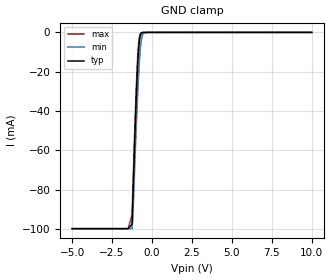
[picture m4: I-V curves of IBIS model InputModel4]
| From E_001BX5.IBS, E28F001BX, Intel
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|*******************Input Model 4************************************
[Model]   InputModel4
Model_type   Input
|   Model for pin A[10]
Vinl = 0.8V
Vinh = 2.0V
|Variable   Typ   Min   Max
C_comp   9.13p   7.20p   11.06p
[Voltage Range]   5.0V   4.5V   5.5V
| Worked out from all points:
|   GND clamp passes 1 mA (typ) near -0.71 V on its own axis
[GND_clamp]
|Voltage   I(typ)   I(min)   I(max)
-5V       -99.85mA   -99.85mA   -99.85mA
-1.5V     -99.85mA   -99.85mA   -99.85mA
-1.25V    -97.6mA    -99.85mA   -93.02mA
-1.2V     -84.57mA   -94.57mA   -79.63mA
-1.05V    -47.49mA   -61.29mA   -42.08mA
-950mV    -25.96mA   -40.81mA   -20.83mA
-850mV    -10.08mA   -23.22mA   -6.469mA
-800mV    -5.085mA   -15.87mA   -2.728mA
-700mV    -816.9uA   -5.687mA   -299.2uA
-600mV    -84.77uA   -1.399mA   -29.88uA
-250mV    0A         0A         0A
10V       0A         0A         0A
[Power_clamp]
| Input buffer circuits of this product do not intrinisically
| require a [Power_clamp] defintion.  This zero current
| [Power_clamp] table is provided for compatibility with
| some IBIS parsers.
|Voltage   I(typ)   I(min)   I(max)
-5V       0A         0A         0A
0V        0A         0A         0A
5V        0A         0A         0A
10V       0A         0A         0A
